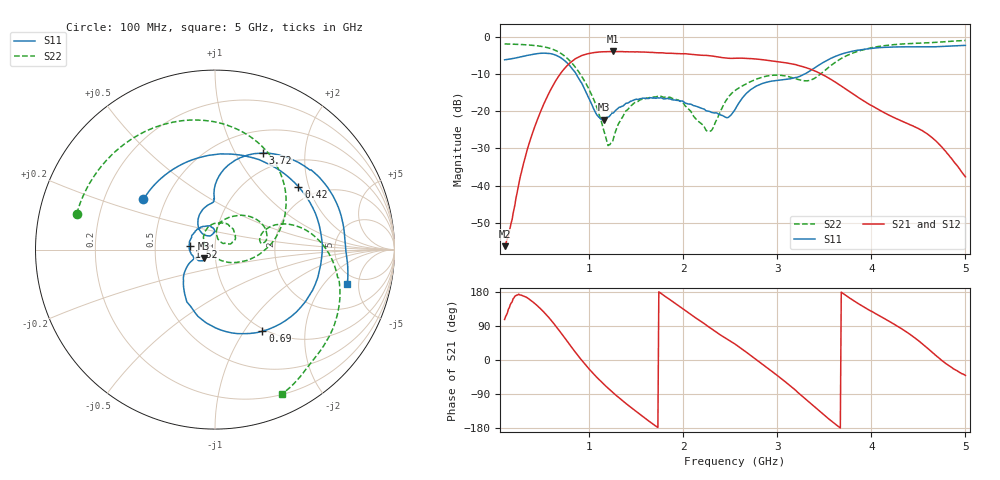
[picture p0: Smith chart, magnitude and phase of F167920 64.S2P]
!  2-Port S-parameters saved by WinCal
! VAR MeasName=S-Parameters (CALIBRATED_DATA) read from VNA (N5242A)
! VAR MeasDate=2016-11-22 9:58:43
! VAR NAME=F167920 64
! VAR FILENAME=F167920 64.S2P
! VAR DATE=2016-11-22 9:58:43
! VAR PHYS_PORTS=1,2
# Hz S DB R 50
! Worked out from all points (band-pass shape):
!   491 points, 100 MHz to 5 GHz, reference 50 ohm
!   highest |S21| = -4.01 dB at 1.25 GHz (marker M1); lowest = -56.3 dB at 100 MHz (marker M2)
!   |S21| within 3 dB of the highest: 798.4 MHz to 3.081 GHz (2.283 GHz wide, 118 % of centre)
!   lowest |S11| = -22.4 dB at 1.16 GHz (marker M3), VSWR 1.17, Z = 44.2 - j4.24 ohm
!   |S11| at or under -10 dB: 858.9 MHz to 3.296 GHz (2.437 GHz wide, 117 % of centre)
!   |S22| runs from -29.3 to -1.1 dB; largest |S21 - S12| = 0.0011
!   S11 on the Smith chart (normalised r, x): 100 MHz: 0.37, +0.28; 420 MHz: 1.61, +1.71; 690 MHz: 0.97, -1.21; 1.52 GHz: 0.75, +0.03; 3.72 GHz: 0.77, +1.30; 5 GHz: 4.01, -3.61
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1e8  -6.25 144.9  -56.29 107.0  -56.72 106.2  -1.98 165.5
2.7e8  -5.45 87.0  -37.29 171.4  -37.45 171.9  -2.13 140.1
4.2e8  -4.70 37.1  -24.25 149.2  -24.26 149.2  -2.41 115.5
5.5e8  -4.51 -8.0  -16.30 117.6  -16.31 117.6  -2.94 90.6
6.9e8  -5.58 -59.9  -10.09 74.8  -10.09 74.9  -4.38 58.8
8.1e8  -8.32 -104.4  -6.76 34.5  -6.75 34.6  -6.96 28.8
9.2e8  -12.51 -138.1  -5.11 -0.6  -5.10 -0.6  -10.74 1.8
1.16e9  -22.35 -141.3  -4.08 -65.3  -4.08 -65.3  -25.63 -76.7
1.25e9  -20.58 -140.6  -4.01 -85.7  -4.00 -85.7  -28.04 -173.7
1.38e9  -18.17 -157.7  -4.10 -112.6  -4.09 -112.6  -20.34 132.0
1.52e9  -16.91 172.8  -4.12 -139.9  -4.12 -139.9  -17.41 100.9
1.74e9  -16.51 134.2  -4.36 179.9  -4.36 179.9  -16.08 65.9
2.03e9  -17.95 99.4  -4.64 129.0  -4.64 129.0  -18.84 25.1
2.27e9  -20.07 92.2  -5.14 87.5  -5.14 87.5  -25.43 51.9
2.55e9  -19.62 126.9  -5.82 42.1  -5.82 42.1  -14.53 68.9
2.88e9  -12.31 103.3  -6.33 -18.3  -6.34 -18.3  -10.66 32.2
3.14e9  -11.33 91.2  -7.27 -68.6  -7.28 -68.7  -10.90 9.3
3.37e9  -8.85 89.8  -8.93 -118.2  -8.94 -118.2  -11.53 16.8
3.72e9  -4.42 63.5  -13.95 171.8  -13.97 171.9  -5.35 9.9
4.19e9  -2.85 25.9  -21.14 102.1  -21.16 102.3  -2.30 -26.8
4.63e9  -2.77 1.6  -26.84 24.0  -26.81 24.2  -1.64 -50.2
5e9  -2.37 -14.4  -37.67 -40.6  -37.72 -39.4  -1.05 -64.9
